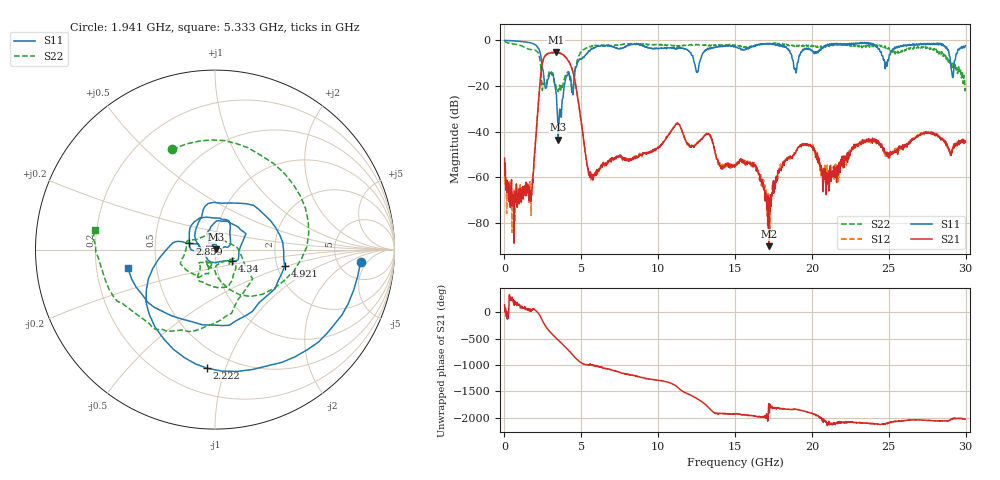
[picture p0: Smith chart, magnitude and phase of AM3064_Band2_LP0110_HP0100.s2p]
# Hz S DB R 50.0
!freq dBS11 angS11 dBS21 angS21 dBS12 angS12 dBS22 angS22
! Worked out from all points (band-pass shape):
!   1600 points, 10 MHz to 29.98 GHz, reference 50 ohm
!   highest |S21| = -5.17 dB at 3.346 GHz (marker M1); lowest = -90.3 dB at 17.22 GHz (marker M2)
!   |S21| within 3 dB of the highest: 2.538 GHz to 4.075 GHz (1.537 GHz wide, 46.5 % of centre)
!   lowest |S11| = -43.5 dB at 3.478 GHz (marker M3), VSWR 1.01, Z = 50.6 + j0.276 ohm
!   |S11| at or under -10 dB: 2.43 GHz to 4.739 GHz (2.31 GHz wide, 64.4 % of centre); 12.35 GHz to 12.67 GHz (320.9 MHz wide, 2.56 % of centre); 18.8 GHz to 19.05 GHz (250.1 MHz wide, 1.32 % of centre)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
!   |S22| runs from -23.5 to -0.2 dB; largest |S21 - S12| = 0.015
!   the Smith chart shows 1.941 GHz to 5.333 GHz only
!   S11 on the Smith chart (normalised r, x): 1.941 GHz: 8.35, -3.37; 2.222 GHz: 0.37, -0.87; 2.859 GHz: 0.75, +0.05; 4.34 GHz: 1.20, -0.15; 4.921 GHz: 2.20, -0.49; 5.333 GHz: 0.34, -0.09
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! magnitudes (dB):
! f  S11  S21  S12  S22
! 10 MHz  0.0  -51.7  -53.8  -0.2
! 553.6 MHz  -0.2  -68.2  -66.8  -1.5
! 1.678 GHz  -1.1  -66.0  -66.2  -4.0
! 1.941 GHz  -1.8  -51.7  -52.2  -4.3
! 2.222 GHz  -3.6  -26.5  -26.3  -5.8
! 2.859 GHz  -16.7  -5.7  -5.7  -15.3
! 3.346 GHz  -22.4  -5.2  -5.3  -20.1
! 3.478 GHz  -43.5  -5.4  -5.4  -21.9
! 4.34 GHz  -18.8  -11.6  -11.4  -18.6
! 4.921 GHz  -8.0  -32.2  -32.3  -5.6
! 5.015 GHz  -8.3  -36.8  -36.7  -5.0
! 5.333 GHz  -6.1  -52.4  -52.7  -3.4
! 10 GHz  -3.6  -47.4  -47.2  -1.9
! 11.27 GHz  -3.5  -36.3  -36.3  -2.5
! 15 GHz  -2.6  -54.9  -54.6  -2.0
! 16.28 GHz  -2.3  -54.6  -55.2  -2.5
! 17.22 GHz  -1.4  -90.3  -76.9  -1.6
! 18.25 GHz  -3.1  -52.7  -52.5  -1.9
! 19.99 GHz  -4.3  -46.5  -46.3  -2.2
! 20.97 GHz  -2.4  -58.1  -62.0  -2.6
! 25 GHz  -8.2  -50.2  -51.3  -3.2
! 29.98 GHz  -2.3  -44.3  -45.1  -20.3
